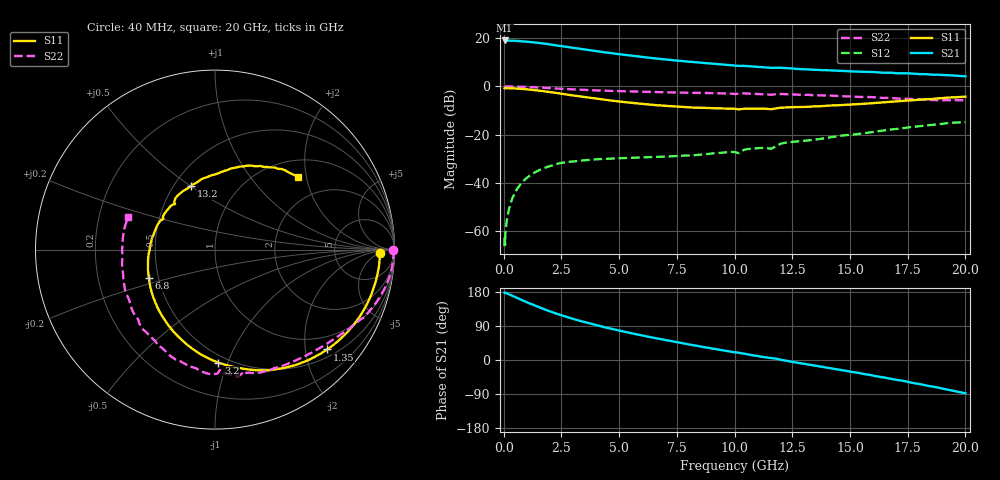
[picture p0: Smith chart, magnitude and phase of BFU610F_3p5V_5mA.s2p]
! Filename:  P:\Prog\Test\Noise\ATS_data\Testdata_Net\SplitFiles\BFU610_2W_A5_HighFreq_3.5V_5mA_D.s2p
! Date/Time: Wed 10/Aug/2011 16:56:36
! BFU610_2W_A5_HighFreq_Bias3_3.5V_1mA_10mA_R.s2p
! MDIF S-parameter v. bias file
! BFU610_2W_A5_HighFreq_3.5V_1mA_10mA
! Date/time Mon Aug 08 14:10:09 2011
! VAR V_out= 3.5000
! VAR I_out= 5.0000
! VAR V_in= 0.8886
! VAR I_in= 0.0396
! Device data file deembeded for feedlines and parallel
! Original file: \SplitFiles\BFU610_2W_A5_HighFreq_3.5V_5mA_R.s2p
! Feed-files: PR003V01_101208_Feed1.s2p, PR003V01_101208_Feed2.s2p
! Parallel-file: PR003V01_101208_Par.s2p
# MHz S MA R 50
!  Freq-MHz  S11-mag  S11-arg  S21-mag  S21-arg  S12-mag  S12-arg  S22-mag  S22-arg
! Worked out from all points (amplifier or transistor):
!   167 points, 40 MHz to 20 GHz, reference 50 ohm
!   highest |S21| = 19.1 dB at 40 MHz (marker M1)
!   |S21| within 3 dB of that: start of sweep to 2.959 GHz
!   unconditionally stable (mu >= 1): 5.369 GHz to 16.49 GHz
!   at 550 MHz: K = 0.04, MSG = 31.0 dB, |S12| = -43.0 dB
!   at 4.2 GHz: K = 0.76, MSG = 22.3 dB, |S12| = -30.2 dB
!   at 20 GHz: K = 0.76, MSG = 9.5 dB, |S12| = -14.8 dB
!   S11 on the Smith chart (normalised r, x): 40 MHz: 22, -5; 1.35 GHz: 0.67, -2.47; 3.2 GHz: 0.44, -0.93; 6.8 GHz: 0.44, -0.17; 13.2 GHz: 0.61, +0.50; 20 GHz: 1.37, +1.78
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40  0.9187 -1.2  8.986 178.0  0.0004842 85.4  0.9929 -0.2
50  0.9118 -1.4  8.944 178.2  0.0007947 48.3  0.9938 -0.4
60  0.9214 -1.6  8.959 177.4  0.000513 83.9  0.9945 -0.5
70  0.9195 -2.1  8.916 177.5  0.0008222 89.9  0.9945 -0.6
140  0.9184 -4.4  8.914 175.9  0.001733 89.8  0.995 -1.6
380  0.9118 -12.1  8.861 169.3  0.004842 86.0  0.9929 -4.5
900  0.8793 -28.4  8.57 155.1  0.01146 75.6  0.9776 -10.7
1350  0.8365 -41.7  8.165 143.6  0.01645 67.3  0.9572 -15.7
1750  0.7924 -52.9  7.734 134.1  0.02022 60.9  0.9363 -19.8
2200  0.7407 -64.8  7.216 124.0  0.0235 55.0  0.9128 -24.1
3200  0.6305 -88.2  6.106 105.1  0.02833 43.5  0.8577 -32.0
3400  0.6109 -92.6  5.921 101.8  0.02903 42.1  0.8495 -33.4
4100  0.5494 -107.1  5.319 90.6  0.03092 37.9  0.8236 -38.1
4900  0.4926 -122.5  4.728 79.0  0.03215 35.0  0.8002 -43.4
5800  0.4426 -139.0  4.192 67.2  0.03331 33.5  0.7788 -49.3
6800  0.4017 -156.6  3.71 55.0  0.03459 33.6  0.7592 -55.7
8600  0.3589 173.7  3.092 34.9  0.03864 37.6  0.7333 -67.6
10200  0.3343 149.3  2.66 19.1  0.04105 42.4  0.7019 -76.9
13200  0.3777 110.7  2.251 -11.9  0.07569 38.0  0.668 -102.4
13400  0.3838 108.3  2.218 -13.9  0.07808 37.2  0.6579 -104.7
16800  0.4835 73.3  1.919 -49.9  0.1278 18.5  0.5719 -143.7
20000  0.6129 41.4  1.62 -87.9  0.1821 -12.9  0.5165 159.1
